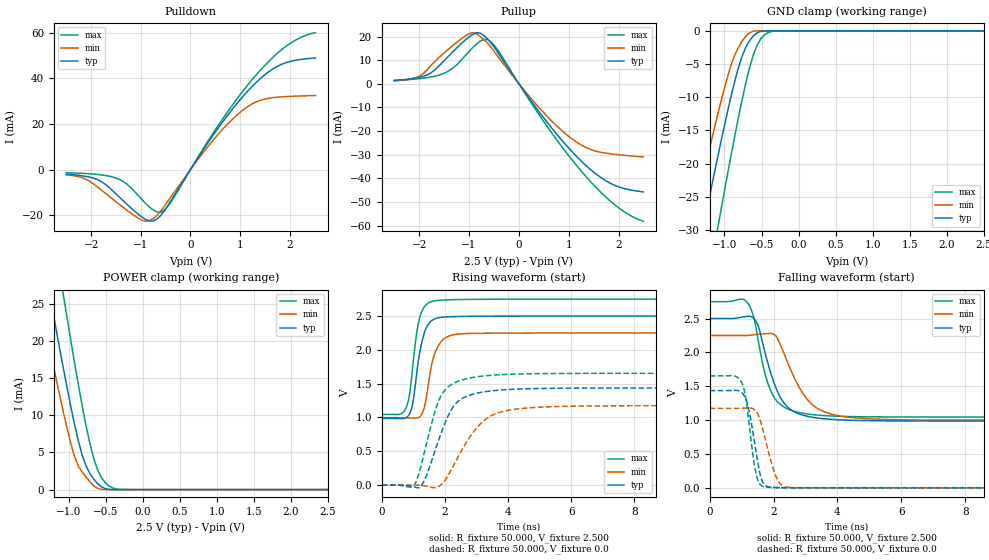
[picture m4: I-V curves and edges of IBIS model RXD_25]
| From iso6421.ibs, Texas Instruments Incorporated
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|   RXD_25 Model
[Model]   RXD_25
Model_type   3-state
| Signals   RXD
Vmeas = 2.2V   |Reference voltage for timing measurements
Cref = 15pF   |Timing specification test load capacitance value
Vref = 0   |Timing specification test load voltage; GND
| variable   typ   min   max
C_comp   2.1pF   1.7pF   2.5pF
|   typ   min   max
[Temperature Range]   25.0   -40   125
[Voltage range]   2.5V   2.25V   2.75V
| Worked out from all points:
|   slope of the pulldown table from 0 to 0.375 V, typ, clamps not added: 30 ohm
|   slope of the pullup table from 0 to 0.375 V, typ, clamps not added: 34 ohm
|   GND clamp passes 1 mA (typ) near -0.63 V on its own axis
|   POWER clamp passes 1 mA (typ) near -0.63 V on its own axis
|   rising waveform, R_fixture 50.000, V_fixture 2.500: 20-80 % time 307ps typ, 332ps min, 273ps max; typ from 0.986 V to 2.5 V
|   rising waveform, R_fixture 50.000, V_fixture 0.0: 20-80 % time 723ps typ, 995ps min, 613ps max; typ from 0 V to 1.44 V
|   falling waveform, R_fixture 50.000, V_fixture 2.500: 20-80 % time 647ps typ, 856ps min, 527ps max; typ from 2.5 V to 0.986 V
|   falling waveform, R_fixture 50.000, V_fixture 0.0: 20-80 % time 312ps typ, 407ps min, 271ps max; typ from 1.44 V to 0 V
[Pulldown]
|Voltage   I(typ)   I(min)   I(max)
-2.5V     -2.011mA   -2.291mA   -1.367mA
-2.12V    -2.917mA   -4.054mA   -1.708mA
-1.816V   -4.979mA   -8.584mA   -2.269mA
-1.36V    -13.53mA   -16.46mA   -5.098mA
-980mV    -20.74mA   -22.15mA   -13.03mA
-752mV    -22.53mA   -21.5mA    -17.65mA
-600mV    -20.16mA   -18.2mA    -18.66mA
-372mV    -12.9mA    -11.28mA   -13.48mA
388mV     12.93mA    11.09mA    13.68mA
1.072V    32.44mA    26.35mA    34.86mA
1.756V    45.32mA    31.74mA    51.1mA
2.516V    48.91mA    32.46mA    60.04mA
[Pullup]
|Voltage   I(typ)   I(min)   I(max)
-2.5V     1.455mA    1.263mA    1.429mA
-1.992V   2.745mA    3.244mA    2.208mA
-1.764V   4.659mA    7.759mA    2.905mA
-1.384V   12.29mA    15.17mA    5.778mA
-1.004V   19.79mA    21.15mA    13.6mA
-776mV    21.44mA    19.99mA    18.07mA
-624mV    18.88mA    17.12mA    18.65mA
-396mV    12.4mA     10.83mA    13.4mA
364mV     -10.73mA   -9.152mA   -11.83mA
1.048V    -28.36mA   -23.07mA   -31.8mA
1.808V    -41.82mA   -29.53mA   -49.2mA
2.492V    -45.74mA   -30.93mA   -58.15mA
[GND_clamp]
|Voltage   I(typ)   I(min)   I(max)
-2.5V     -98.72mA   -81.59mA   -121.6mA
-1.48V    -40.39mA   -31.08mA   -54.46mA
-1.429V   -37.53mA   -28.6mA    -51.16mA
-1.276V   -29.02mA   -21.23mA   -41.34mA
-1.072V   -17.97mA   -11.73mA   -28.49mA
-868mV    -7.877mA   -3.834mA   -16.23mA
-766mV    -3.954mA   -1.633mA   -10.58mA
-664mV    -1.515mA   -327.9uA   -5.663mA
-562mV    -316.6uA   -9.583uA   -2.218mA
-511mV    -91.87uA   -874.4nA   -1.22mA
-358mV    -477.6nA   -336.4pA   -95.12uA
2.5V      0A         0A         -1.714nA
[POWER_clamp]
|Voltage   I(typ)   I(min)   I(max)
-2.5V     97.95mA    81mA       120.7mA
-1.427V   35.94mA    27.33mA    49.01mA
-1.376V   33.06mA    24.84mA    45.68mA
-1.274V   27.35mA    19.9mA     39.07mA
-1.223V   24.53mA    17.46mA    35.79mA
-1.07V    16.26mA    10.38mA    26.14mA
-917mV    8.63mA     4.356mA    16.89mA
-815mV    4.575mA    2.345mA    11.17mA
-611mV    828.2uA    171.4uA    2.709mA
-458mV    35.84uA    324.5nA    506.8uA
-305mV    214.3nA    118.4pA    31uA
2.5V      0A         0A         0A
[Ramp]
| variable   typ   min   max
dV/dt_r   0.862/0.723n   0.705/0.995n   0.992/0.613n
dV/dt_f   0.908/0.647n   0.752/0.855n   1.023/0.527n
R_load = 50.000
[Rising Waveform]
R_fixture= 50.000
V_fixture= 2.500
V_fixture_min= 2.250
V_fixture_max= 2.750
|time   V(typ)   V(min)   V(max)
0s        986.3mV    997.3mV    1.045V
646ps     983.4mV    997.3mV    1.064V
874ps     1.048V     995mV      1.326V
995ps     1.245V     992.1mV    1.808V
1.185ns   1.912V     1.004V     2.446V
1.354ns   2.257V     1.157V     2.64V
1.628ns   2.446V     1.869V     2.72V
1.918ns   2.482V     2.142V     2.735V
2.478ns   2.494V     2.236V     2.744V
15ns      2.5V       2.25V      2.75V
[Rising Waveform]
R_fixture= 50.000
V_fixture= 0.0
V_fixture_min= 0.0
V_fixture_max= 0.0
|time   V(typ)   V(min)   V(max)
0s        318.7nV    205.6nV    910.5nV
973ps     -20.34mV   404uV      -23.57mV
1.244ns   -13.53mV   -5.275mV   285.5mV
1.633ns   429.8mV    -36.79mV   999.5mV
1.873ns   756.9mV    2.536mV    1.315V
2.272ns   1.162V     287.5mV    1.504V
2.694ns   1.314V     642.8mV    1.574V
3.433ns   1.391V     1.016V     1.623V
4.614ns   1.425V     1.141V     1.646V
15ns      1.436V     1.175V     1.653V
[Falling Waveform]
R_fixture= 50.000
V_fixture= 2.500
V_fixture_min= 2.250
V_fixture_max= 2.750
|time   V(typ)   V(min)   V(max)
0s        2.5V       2.25V      2.75V
1.056ns   2.525V     2.249V     2.784V
1.394ns   2.495V     2.261V     2.495V
1.699ns   2.061V     2.274V     1.752V
1.939ns   1.656V     2.278V     1.405V
2.277ns   1.288V     2.042V     1.209V
2.739ns   1.103V     1.54V      1.119V
3.399ns   1.03V      1.166V     1.074V
4.549ns   996.2mV    1.034V     1.052V
15ns      986.3mV    997.3mV    1.045V
[Falling Waveform]
R_fixture= 50.000
V_fixture= 0.0
V_fixture_min= 0.0
V_fixture_max= 0.0
|time   V(typ)   V(min)   V(max)
0s        1.436V     1.175V     1.653V
756ps     1.439V     1.175V     1.655V
1.011ns   1.404V     1.176V     1.545V
1.201ns   1.207V     1.179V     1.078V
1.452ns   532.5mV    1.13V      207.2mV
1.582ns   196.6mV    995.7mV    49.68mV
1.709ns   49.7mV     776.8mV    15.91mV
2.099ns   4.094mV    143.2mV    3.598mV
2.429ns   1.805mV    9.509mV    1.764mV
15ns      741.6pV    1.136nV    139.2nV
